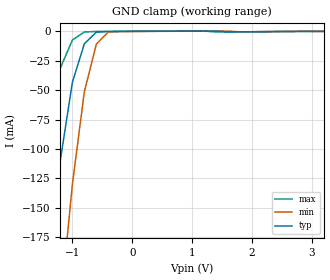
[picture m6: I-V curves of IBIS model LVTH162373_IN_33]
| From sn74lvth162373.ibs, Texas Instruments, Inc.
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|   Model LVTH162373 Input_IN_33
[Model]   LVTH162373_IN_33
Model_type  Input
Polarity   Inverting
Vinl = 0.8V
Vinh = 2.0V
| variable   typ   min   max
C_comp   3p   NA   NA
[Temperature Range]   25   -40   85
[Voltage range]   3.3   3.0   3.6
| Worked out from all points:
|   GND clamp passes 1 mA (typ) near -0.61 V on its own axis
|Process range|   weak   strong
[GND Clamp]
|   Voltage   I(typ)   I(min)   I(max)
-5V       -1.85A     -2.21A     -1.58A
-1.8V     -384mA     -546mA     -244mA
-1.6V     -292mA     -442mA     -160mA
-1.4V     -201mA     -338mA     -80.1mA
-1.2V     -109mA     -234mA     -31mA
-1V       -43.2mA    -130mA     -7.29mA
-800mV    -10.5mA    -51.1mA    -519uA
-600mV    -674uA     -10.8mA    -78.8uA
-400mV    -113uA     -524uA     -25.2uA
1.2V      239uA      233uA      236uA
1.4V      224uA      253uA      -480uA
3.2V      -97.6pA    828nA      -618pA
